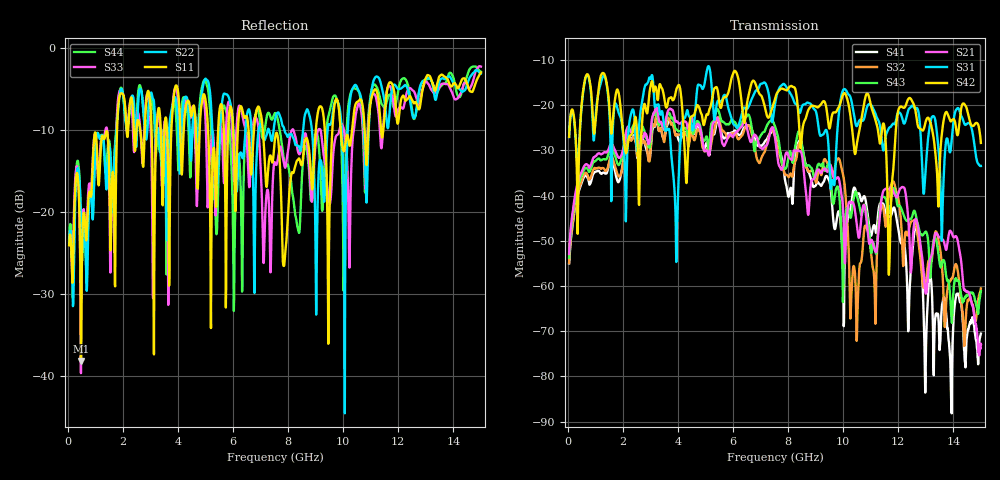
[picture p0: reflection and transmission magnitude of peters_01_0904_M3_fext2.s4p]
# MHZ S RI R 50.00
! FREQ  S11  S12  S13  S14
!  S21  S22  S23  S24
!  S31  S32  S33  S34
!  S41  S42  S43  S44
!  REAL  IMAG  REAL  IMAG  REAL  IMAG  REAL  IMAG
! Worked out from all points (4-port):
!   1496 points, 50 MHz to 15 GHz, reference 50 ohm
!   strongest paths, dB at 50 MHz, 3.79 GHz, 7.53 GHz, 11.27 GHz, 15 GHz:
!     S42: -27.0, -18.6, -18.5, -25.8, -28.3
!     S31: -27.0, -32.8, -19.6, -23.3, -33.4
!     S21: -52.9, -21.0, -27.4, -48.6, -72.9
!     S43: -53.7, -22.8, -24.7, -47.4, -61.1
!     S32: -54.9, -24.1, -27.0, -47.3, -60.5
!     S41: -55.0, -24.0, -26.8, -43.9, -70.5
!   lowest |S11| = -38.2 dB at 480 MHz (marker M1), VSWR 1.02, Z = 49.1 + j0.852 ohm
!   |S11| at or under -10 dB: start of sweep to 1.79 GHz; 7.083 GHz to 9.007 GHz (1.924 GHz wide, 23.9 % of centre); 9.909 GHz to 10.32 GHz (413.7 MHz wide, 4.09 % of centre)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
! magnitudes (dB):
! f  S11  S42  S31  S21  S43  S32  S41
! 50 MHz  -24.1  -27.0  -27.0  -52.9  -53.7  -54.9  -55.0
! 480 MHz  -38.2  -21.7  -22.1  -35.0  -35.9  -37.1  -37.6
! 7.43 GHz  -14.0  -20.5  -23.7  -24.8  -23.4  -25.4  -25.4
! 10.5 GHz  -6.6  -28.4  -24.6  -46.8  -40.0  -71.2  -39.6
! 11.68 GHz  -4.2  -54.8  -24.9  -38.5  -43.6  -39.1  -44.7
! 12.07 GHz  -6.9  -20.4  -21.8  -38.4  -42.3  -43.7  -49.9
! 15 GHz  -3.0  -28.3  -33.4  -72.9  -61.1  -60.5  -70.5
